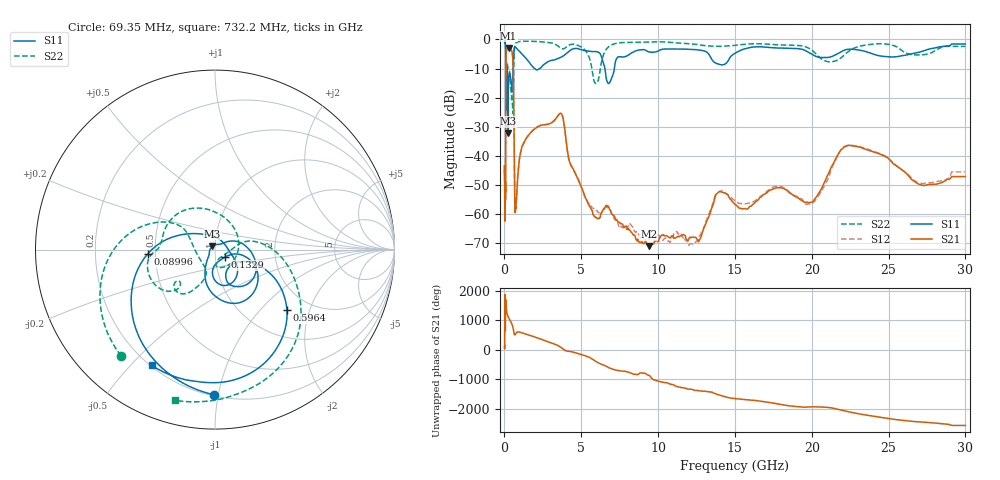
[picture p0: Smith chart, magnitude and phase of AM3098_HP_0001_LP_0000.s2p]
! Date/Time: Thu, Feb 28, 2019 8:31 AM
! Network Analyzer: Agilent Technologies E8364B Rev: A.07.50.67
! Sweep from 0.010 to 30.000 GHz, 1601 Points, Sweep Type: LOG
! Power Supply: 5.023 V, 0.002 A
# Hz S DB R 50
!freq MagS11 AngS11 MagS21 AngS21 MagS12 AngS12 MagS22 AngS22
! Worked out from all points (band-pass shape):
!   1601 points, 10 MHz to 30 GHz, reference 50 ohm
!   highest |S21| = -2.94 dB at 267.8 MHz (marker M1); lowest = -71.1 dB at 9.396 GHz (marker M2)
!   |S21| within 3 dB of the highest: 104.7 MHz to 533.6 MHz (428.9 MHz wide, 134 % of centre)
!   lowest |S11| = -32.3 dB at 228.2 MHz (marker M3), VSWR 1.05, Z = 48.6 + j1.94 ohm
!   |S11| at or under -10 dB: 175.9 MHz to 562.1 MHz (386.1 MHz wide, 105 % of centre); 1.958 GHz to 2.277 GHz (318.9 MHz wide, 15.1 % of centre); 6.535 GHz to 7.153 GHz (617.2 MHz wide, 9.02 % of centre)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
!   |S22| runs from -25.5 to -0.6 dB; largest |S21 - S12| = 0.011
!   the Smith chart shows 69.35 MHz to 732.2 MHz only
!   S11 on the Smith chart (normalised r, x): 69.35 MHz: 0.21, -0.97; 89.96 MHz: 0.45, -0.02; 132.9 MHz: 1.12, -0.09; 596.4 MHz: 1.53, -1.43; 732.2 MHz: 0.20, -0.57
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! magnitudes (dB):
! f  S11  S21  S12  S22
! 10 MHz  -0.3  -43.5  -45.0  -0.6
! 38.04 MHz  -0.5  -59.8  -58.9  -0.8
! 69.35 MHz  -1.8  -53.3  -51.7  -2.1
! 89.96 MHz  -8.5  -18.0  -17.9  -10.6
! 98.93 MHz  -24.3  -7.7  -7.7  -17.3
! 132.9 MHz  -23.1  -3.7  -3.7  -11.5
! 144.7 MHz  -13.6  -3.5  -3.4  -10.2
! 187.7 MHz  -11.6  -3.3  -3.3  -8.3
! 228.2 MHz  -32.3  -3.0  -3.0  -10.0
! 267.8 MHz  -14.9  -2.9  -2.9  -10.5
! 550.5 MHz  -11.9  -7.2  -7.2  -25.3
! 596.4 MHz  -5.6  -17.1  -17.0  -10.9
! 665.8 MHz  -2.6  -55.0  -55.5  -2.3
! 732.2 MHz  -2.7  -58.1  -57.7  -1.2
! 2.084 GHz  -10.4  -30.3  -30.3  -0.7
! 3.686 GHz  -6.1  -25.5  -25.4  -3.1
! 5.959 GHz  -4.2  -61.2  -58.8  -15.2
! 7.926 GHz  -5.8  -64.3  -64.4  -1.0
! 9.396 GHz  -4.2  -71.1  -68.9  -0.9
! 19.8 GHz  -4.5  -56.2  -56.6  -3.0
! 22.67 GHz  -3.4  -36.6  -36.5  -3.2
! 30 GHz  -1.6  -47.2  -45.6  -2.4
